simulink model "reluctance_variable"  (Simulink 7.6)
settings: Solver=ode23tb  StartTime=0.0  StopTime=10  RelTol=1e-3
InitFcn:
  | a=1% %0.8;
StopFcn:
  | close all, clc
  | load  reluctance_flux.mat
  | plotyy(x(1,:),x(2,:),x(1,:),x(3,:))
  | grid
  | title('Flux et reluctance')
  | xlabel('temps')
undefined symbols (not defined in the file or in its folder): sinc
libraries: fl_lib x5, nesl_utility x4

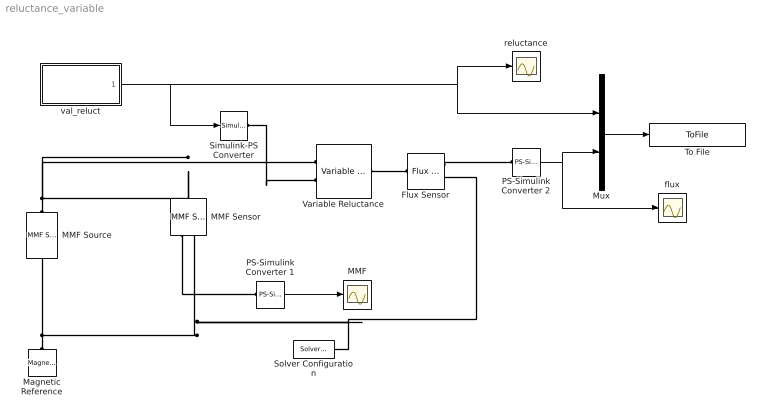
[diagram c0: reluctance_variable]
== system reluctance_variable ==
  Flux Sensor : fl_lib/Magnetic/Magnetic Sensors/Flux Sensor  DialogController=NetworkEngine.DynNeDlgSource  SystemSampleTime=-1  phi_Log=off  mmf_Log=off  LocalVarNames=|phi|mmf  LocalVarDescs=|phi|mmf  LocalVarLogging=[0 0]
  MMF : Scope
  MMF Sensor : fl_lib/Magnetic/Magnetic Sensors/MMF Sensor  DialogController=NetworkEngine.DynNeDlgSource  SystemSampleTime=-1  phi_Log=off  mmf_Log=off  LocalVarNames=|phi|mmf  LocalVarDescs=|phi|mmf  LocalVarLogging=[0 0]
  MMF Source : fl_lib/Magnetic/Magnetic Sources/MMF Source  DialogController=NetworkEngine.DynNeDlgSource  SystemSampleTime=-1  mmf0=1 A  phi_Log=off  mmf_Log=off  LocalVarNames=|phi|mmf  LocalVarDescs=|phi|mmf  LocalVarLogging=[0 0]
  Magnetic Reference : fl_lib/Magnetic/Magnetic Elements/Magnetic Reference  DialogController=NetworkEngine.DynNeDlgSource  SystemSampleTime=-1  phi_Log=off  LocalVarNames=|phi  LocalVarDescs=|phi  LocalVarLogging=0
  Mux : Mux  Inputs=2
  PS-Simulink Converter 1 : nesl_utility/PS-Simulink Converter  DialogController=NetworkEngine.DynNeUtilDlgSource  SystemSampleTime=-1  PhysicalDomain=network_engine_domain  LeftPortType=input  RightPortType=output  SubClassName=ps_output  Unit=1  AffineConversion=off
  PS-Simulink Converter 2 : nesl_utility/PS-Simulink Converter  DialogController=NetworkEngine.DynNeUtilDlgSource  SystemSampleTime=-1  PhysicalDomain=network_engine_domain  LeftPortType=input  RightPortType=output  SubClassName=ps_output  Unit=1  AffineConversion=off
  Simulink-PS Converter : nesl_utility/Simulink-PS Converter  DialogController=NetworkEngine.DynNeUtilDlgSource  SystemSampleTime=-1  PhysicalDomain=network_engine_domain  LeftPortType=input  RightPortType=output  SubClassName=ps_input  Unit=1  AffineConversion=off  InputFilterTimeConstant=.001  UdotUserProvided=0
  Solver Configuration : nesl_utility/Solver Configuration  DialogController=NetworkEngine.DynNeUtilDlgSource  SystemSampleTime=-1  PhysicalDomain=network_engine_domain  LeftPortType=input  RightPortType=generic  SubClassName=solver  Accelerate=off  Profile=off  ResidualTolerance=1e-9  MaxNonlinIter=3  MaxModeIter=2  DoFixedCost=off  UseLocalSampling=off  DoDC=off  LinearAlgebra=Sparse  LocalSolverSampleTime=.001  LocalSolverChoice=NE_BACKWARD_EULER_ADVANCER  UseLocalSolver=off
  To File : ToFile  Filename=reluctance_flux  MatrixName=x
  Variable Reluctance : fl_lib/Magnetic/Magnetic Elements/Variable Reluctance  DialogController=NetworkEngine.DynNeDlgSource  SystemSampleTime=-1  Xmin=5 mm  CSA=0.01 m^2  mur=1  phi_Log=off  mmf_Log=off  LocalVarNames=|phi|mmf  LocalVarDescs=|phi|mmf  LocalVarLogging=[0 0]
  flux : Scope
  reluctance : Scope
  val_reluct : Subsystem
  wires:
  PS-Simulink Converter 2/1 -> Mux/2, flux/1
  PS-Simulink Converter 1/1 -> MMF/1
  val_reluct/1(R) -> Simulink-PS Converter/1, Mux/1, reluctance/1
  Mux/1 -> To File/1
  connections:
  MMF Source/LConn1 -- MMF Sensor/LConn1 -- Variable Reluctance/LConn1
  Variable Reluctance/RConn1 -- Flux Sensor/LConn1
  Magnetic Reference/LConn1 -- Flux Sensor/RConn2 -- Solver Configuration/RConn1 -- MMF Sensor/RConn2 -- MMF Source/RConn1
  Simulink-PS Converter/RConn1 -- Variable Reluctance/LConn2
  Flux Sensor/RConn1 -- PS-Simulink Converter 2/LConn1
  MMF Sensor/RConn1 -- PS-Simulink Converter 1/LConn1

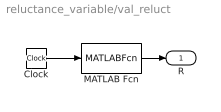
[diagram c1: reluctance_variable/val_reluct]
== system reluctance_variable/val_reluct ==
  Clock : Clock
  MATLAB Fcn : MATLABFcn  MATLABFcn=sinc(u)+2
  R : Outport
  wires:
  Clock/1 -> MATLAB Fcn/1
  MATLAB Fcn/1 -> R/1
